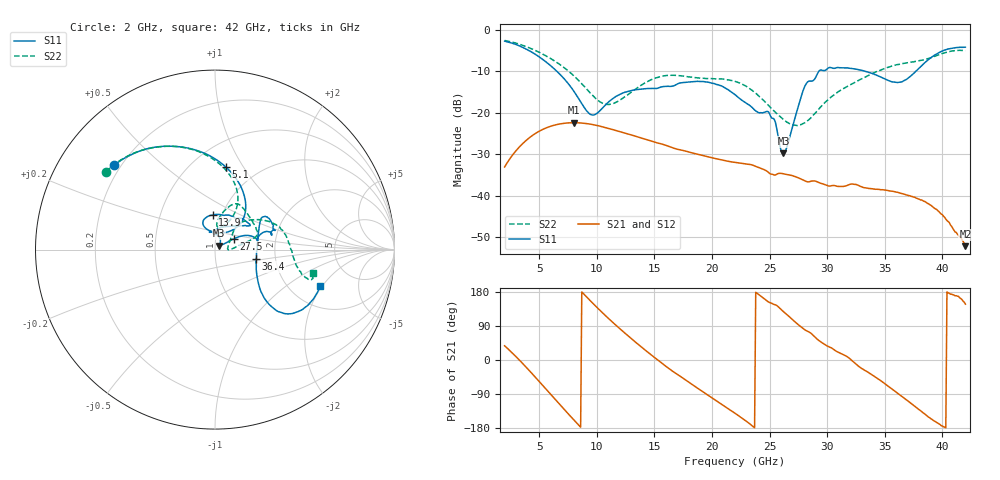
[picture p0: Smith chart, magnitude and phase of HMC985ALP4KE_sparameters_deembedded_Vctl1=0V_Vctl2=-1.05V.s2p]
!s2p File: Measurements: S11, S21, S12, S22
# GHz S dB R 50.0
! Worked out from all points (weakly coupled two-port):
!   401 points, 2 GHz to 42 GHz, reference 50 ohm
!   highest |S21| = -22.38 dB at 8 GHz (marker M1); lowest = -52.2 dB at 42 GHz (marker M2)
!   lowest |S11| = -29.8 dB at 26.2 GHz (marker M3), VSWR 1.07, Z = 52.4 + j2.27 ohm
!   |S11| at or under -10 dB: 6.551 GHz to 29.27 GHz (22.72 GHz wide, 127 % of centre); 33.35 GHz to 37.7 GHz (4.346 GHz wide, 12.2 % of centre)
!   |S22| runs from -23.1 to -2.5 dB; largest |S21 - S12| = 0.00014
!   S11 on the Smith chart (normalised r, x): 2 GHz: 0.17, +0.35; 5.1 GHz: 0.72, +0.84; 13.9 GHz: 0.90, +0.36; 27.5 GHz: 1.22, +0.15; 36.4 GHz: 1.58, -0.18; 42 GHz: 2.90, -1.91
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2  -2.69 140.2  -33.07 37.5  -33.08 37.5  -2.52 144.4
3.5  -4.11 112.5  -27.62 -7.0  -27.61 -7.0  -3.63 120.0
5.1  -6.68 82.4  -24.29 -60.0  -24.30 -60.0  -5.52 95.4
8  -14.73 45.7  -22.38 -157.8  -22.39 -157.8  -11.03 63.5
8.7  -17.80 51.8  -22.47 179.6  -22.47 179.6  -12.98 61.7
9.7  -20.53 85.6  -22.86 148.4  -22.86 148.4  -15.97 66.1
10.9  -17.69 113.7  -23.66 112.9  -23.66 112.9  -17.97 80.0
13.9  -14.25 93.9  -26.10 33.6  -26.10 33.7  -13.25 77.2
15.4  -13.94 73.0  -27.35 -2.2  -27.36 -2.2  -11.33 68.4
19.4  -12.52 34.6  -30.45 -87.7  -30.46 -87.7  -11.69 36.2
22  -15.61 52.2  -31.95 -140.5  -31.96 -140.5  -12.40 17.6
25  -20.19 97.9  -34.63 151.6  -34.64 151.6  -18.48 7.4
26.2  -29.80 41.9  -34.73 127.8  -34.72 127.7  -21.60 -0.2
27.5  -18.40 29.7  -35.71 93.0  -35.71 92.8  -22.96 5.6
28.1  -13.36 20.7  -36.47 78.9  -36.49 78.8  -22.32 16.2
28.7  -12.31 12.9  -36.45 67.7  -36.45 67.7  -20.85 27.0
31  -9.08 23.3  -37.76 19.9  -37.76 19.7  -14.83 47.5
33.3  -9.96 34.4  -38.10 -27.7  -38.12 -27.7  -11.38 38.0
35.4  -12.27 12.3  -38.85 -71.5  -38.81 -71.7  -8.93 23.8
36.4  -12.57 -12.8  -39.42 -94.2  -39.42 -94.3  -8.15 16.0
39.5  -5.80 -43.3  -43.30 -164.4  -43.38 -164.5  -6.14 -14.5
42  -4.14 -19.1  -52.19 147.5  -52.42 146.5  -5.01 -13.3
